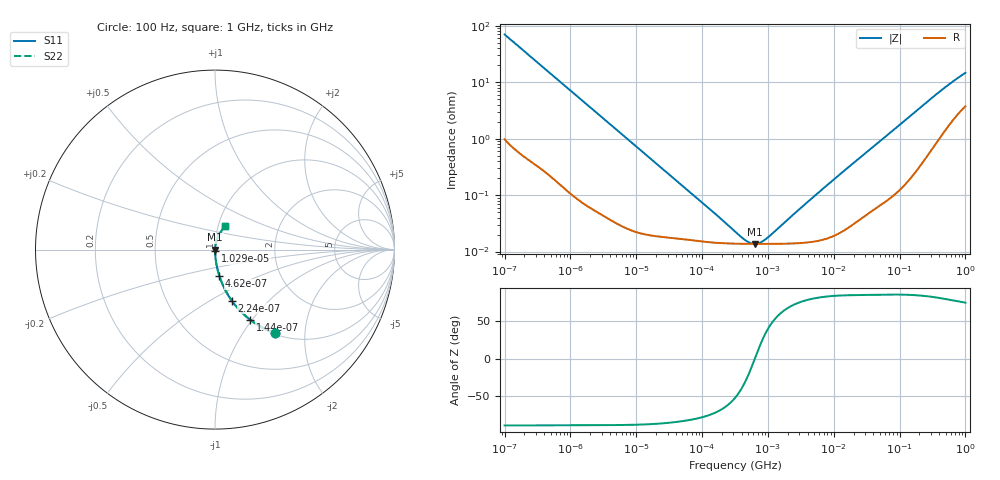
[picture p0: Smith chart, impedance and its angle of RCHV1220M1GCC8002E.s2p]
! RCHV1220M1GCC8002E  S-PARAMETER MODEL  (AEC-Q200 qualified)
! Model Generated by ELNA Corporation (http://www.ty-top.com)
! Version 1.0
! ELNA Control No. 240229
! Copyright (c) 2024 ELNA CO.,LTD. All Rights Reserved.
! Products Name : CONDUCTIVE POLYMER HYBRID ALUMINUM ELECTROLYTIC CAPACITORS
! Characteristics :
!  Capacitance  :  22uF  ,  Rated voltage  :  35V
!  Operating Temp. Range  :  -55 to +105 degC  ,  Endurance  :  10000hr at 105 degC
!  Dimension D  :  5mm  ,  Dimension L  :  5.8mm
! Frequency Range : 100Hz - 1GHz
! External Node Assignments :
!  1  o---| |---o  2
# MHz S RI R 50
!Freq[MHz].  S11 Real  S11 Imag  S21 Real  S21 Imag  S12 Real  S12 Imag  S22 Real  S22 Imag
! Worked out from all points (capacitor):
!   401 points, 100 Hz to 1 GHz, reference 50 ohm
!   read as one part in series: C = 22.7 uF near 108 Hz
!   lowest |Z| = 13.6 mohm at 627.3 kHz (marker M1)
!   series resonance near 631.2 kHz, so ESL is about 2.8 nH
!   S11 on the Smith chart (normalised r, x): 100 Hz: 1.02, -1.40; 144 Hz: 1.01, -0.98; 224 Hz: 1.01, -0.63; 462 Hz: 1.00, -0.31; 10.29 kHz: 1.00, -0.01; 1 GHz: 1.07, +0.28
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0.0001  0.3315 -0.4638  0.6685 0.4638  0.6685 0.4638  0.3315 -0.4638
0.000144  0.1955 -0.3901  0.8045 0.3901  0.8045 0.3901  0.1955 -0.3901
0.000224  0.0929 -0.2836  0.9071 0.2836  0.9071 0.2836  0.0929 -0.2836
0.000309  0.0523 -0.2154  0.9477 0.2154  0.9477 0.2154  0.0523 -0.2154
0.000462  0.025 -0.1489  0.975 0.1489  0.975 0.1489  0.025 -0.1489
0.000781  0.00955 -0.0901  0.9905 0.0901  0.9905 0.0901  0.00955 -0.0901
0.001488  0.00304 -0.0479  0.997 0.0479  0.997 0.0479  0.00304 -0.0479
0.010292  0.000268 -0.00704  0.9997 0.00704  0.9997 0.00704  0.000268 -0.00704
0.022131  0.000194 -0.00328  0.9998 0.00328  0.9998 0.00328  0.000194 -0.00328
0.12517  0.000147 -0.000574  0.9999 0.000574  0.9999 0.000574  0.000147 -0.000574
0.316228  0.000138 -0.000179  0.9999 0.000179  0.9999 0.000179  0.000138 -0.000179
0.473151  0.000137 -6.99e-05  0.9999 6.99e-05  0.9999 6.99e-05  0.000137 -6.99e-05
0.555904  0.000136 -3.05e-05  0.9999 3.05e-05  0.9999 3.05e-05  0.000136 -3.05e-05
0.627336  0.000136 -1.46e-06  0.9999 1.46e-06  0.9999 1.46e-06  0.000136 -1.46e-06
0.767361  0.000136 4.71e-05  0.9999 -4.71e-05  0.9999 -4.71e-05  0.000136 4.71e-05
0.977237  0.000136 0.000108  0.9999 -0.000108  0.9999 -0.000108  0.000136 0.000108
4.704354  0.000149 0.000875  0.9999 -0.000875  0.9999 -0.000875  0.000149 0.000875
69.9842  0.00101 0.0123  0.999 -0.0123  0.999 -0.0123  0.00101 0.0123
184.0772  0.00375 0.0316  0.9962 -0.0316  0.9962 -0.0316  0.00375 0.0316
395.8221  0.0138 0.0642  0.9862 -0.0642  0.9862 -0.0642  0.0138 0.0642
695.825  0.0336 0.1011  0.9664 -0.1011  0.9664 -0.1011  0.0336 0.1011
1000  0.0537 0.1292  0.9463 -0.1292  0.9463 -0.1292  0.0537 0.1292
